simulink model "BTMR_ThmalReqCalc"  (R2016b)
settings: Solver=FixedStepDiscrete  StartTime=0.0  StopTime=10.0  FixedStep=0.1  RelTol=1e-3  EnableMultiTasking=on
undefined symbols (not defined in the file or in its folder): BMS_cntThmStbNum_C, BTMR_cntThmalReqVal_C, BTMR_flgCoolPwrCal_C, BTMR_pChrgClntPwrLv1_C, BTMR_pChrgClntPwrLv2_C, BTMR_pChrgClntPwrLv3_C, BTMR_pChrgClntPwrLv4_C, BTMR_pChrgClntPwrLv5_C, BTMR_pChrgClntPwrLv6_C, BTMR_pCoolPwrVal_C, BTMR_pHtgACPwrReq_C, BTMR_pHtgDCPwrReq_C, BTMR_pHtgDrvPwrReq_C, BTMR_pHtgsStage1_CUR, BTMR_pHtgsStage2_CUR, BTMR_pNormClntPwrLv1_C, BTMR_pNormClntPwrLv2_C, BTMR_pNormClntPwrLv3_C, BTMR_r861BrsDrvSoc_C, BTMR_r861HtgDrvSoc_C, BTMR_r891BrsDrvSoc_C, BTMR_r891HtgDrvSoc_C, BTMR_rCoolClbFlg_C, BTMR_rFlashClbFlg_C, BTMR_rHeatClbFlg_C, BTMR_t861BrsDiffLv0Temp_C, BTMR_t861BrsDiffLv1Temp_C, BTMR_t861CoolChrgAces2Temp_C, BTMR_t861CoolChrgAces3Temp_C, BTMR_t861CoolChrgAcesTemp_C, BTMR_t861CoolChrgDiffDebTemp_C, BTMR_t861CoolChrgEndDiffTemp_C, BTMR_t861CoolChrgExitLv2Temp_C, BTMR_t861CoolChrgExitLv3Temp_C, BTMR_t861CoolChrgExitTemp_C, BTMR_t861CoolChrgIntLv0Temp_C, BTMR_t861CoolChrgIntLv1Temp_C, BTMR_t861CoolChrgIntLv2Temp_C, BTMR_t861CoolChrgIntLv3Temp_C, BTMR_t861CoolChrgIntLv4Temp_C, BTMR_t861CoolChrgIntLv5Temp_C, BTMR_t861CoolDCDebTemp_C, BTMR_t861CoolNormAcesTemp_C, BTMR_t861CoolNormDiffDebTemp_C, BTMR_t861CoolNormEndDiffTemp_C, BTMR_t861CoolNormExitLv2Temp_C, BTMR_t861CoolNormExitLv3Temp_C, BTMR_t861CoolNormExitTemp_C, BTMR_t861CoolNormIntLv0Temp_C, BTMR_t861CoolNormIntLv1Temp_C, BTMR_t861CoolNormLv2Temp_C, BTMR_t861CoolNormLv3Temp_C, BTMR_t861HtgACDiffDebTemp_C, BTMR_t861HtgACEndDiffTemp_C, BTMR_t861HtgACStartHiTemp_C, BTMR_t861HtgACStartLoTemp_C, BTMR_t861HtgACStopTemp_C, BTMR_t861HtgDCDiffDebTemp_C, BTMR_t861HtgDCEndDiffTemp_C, BTMR_t861HtgDCIntLv0Temp_C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
libraries: AIWAYS_Powertrain_BMS_lib x78, simulink x9
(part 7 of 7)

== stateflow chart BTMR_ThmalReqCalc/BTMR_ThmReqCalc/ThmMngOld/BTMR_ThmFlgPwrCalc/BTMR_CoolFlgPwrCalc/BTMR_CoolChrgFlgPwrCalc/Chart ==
  state CoolChrgDefault
    en:
    BTMR_stsClntStg=enmThmCoolChrgStg_861.Default;
  state CoolChrgStage1
    state CoolChrgStage1Norm
      en:
      BTMR_stsClntStg=enmThmCoolChrgStg_861.Stg_Lv1Res;
    state CoolChrgStage1Reduce
      en:
      BTMR_stsClntStg=enmThmCoolChrgStg_861.Stg_Lv1Red;
    (default) -> CoolChrgStage1Norm
    CoolChrgStage1Norm -> CoolChrgStage1Reduce : [ CoolChrgStage1PowRed ]
    CoolChrgStage1Reduce -> CoolChrgStage1Norm : [ CoolChrgStage1PowRes ]
  state CoolChrgStage2
    state CoolChrgStage2Norm
      en:
      BTMR_stsClntStg=enmThmCoolChrgStg_861.Stg_Lv2Res;
    state CoolChrgStage2Reduce
      en:
      BTMR_stsClntStg=enmThmCoolChrgStg_861.Stg_Lv2Red;
    (default) -> CoolChrgStage2Norm
    CoolChrgStage2Norm -> CoolChrgStage2Reduce : [ CoolChrgStage2PowRed ]
    CoolChrgStage2Reduce -> CoolChrgStage2Norm : [ CoolChrgStage2PowRes ]
  state CoolChrgStage3
    state CoolChrgStage3Norm
      en:
      BTMR_stsClntStg=enmThmCoolChrgStg_861.Stg_Lv3Res;
    state CoolChrgStage3Reduce
      en:
      BTMR_stsClntStg=enmThmCoolChrgStg_861.Stg_Lv3Red;
    (default) -> CoolChrgStage3Norm
    CoolChrgStage3Norm -> CoolChrgStage3Reduce : [ CoolChrgStage3PowRed ]
    CoolChrgStage3Reduce -> CoolChrgStage3Norm : [ CoolChrgStage3PowRes ]
  (default) -> CoolChrgDefault
  CoolChrgDefault -> CoolChrgStage1
  CoolChrgStage1 -> CoolChrgStage2 : [ CoolChrgStage2Ena ]
  CoolChrgStage2 -> CoolChrgStage1 : [ CoolChrgStage2Ext ]
  CoolChrgStage2 -> CoolChrgStage3 : [ CoolChrgStage3Ena ]
  CoolChrgStage3 -> CoolChrgStage2 : [ CoolChrgStage3Ext ]
  data: CoolChrgStage2Ena input; CoolChrgStage3Ena input; BTMR_stsClntStg output Enum: enmThmCoolChrgStg_861; BTMR_pChrgClntPwrLv1_C parameter; BTMR_pChrgClntPwrLv2_C parameter; BTMR_pChrgClntPwrLv3_C parameter; CoolChrgStage2Ext input; CoolChrgStage3Ext input; CoolChrgStage1PowRed input; CoolChrgStage1PowRes input; CoolChrgStage2PowRed input; CoolChrgStage2PowRes input; CoolChrgStage3PowRed input; CoolChrgStage3PowRes input; BTMR_pChrgClntPwrLv4_C parameter; BTMR_pChrgClntPwrLv5_C parameter; BTMR_pChrgClntPwrLv6_C parameter

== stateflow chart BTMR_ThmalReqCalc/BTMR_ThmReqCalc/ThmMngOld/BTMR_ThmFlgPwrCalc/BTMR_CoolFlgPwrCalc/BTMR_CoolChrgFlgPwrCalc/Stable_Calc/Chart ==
  state Default_Stt
    en:
    i=uint8(0);
    flg_out=false;
  state AddCourse_Stt
    en:
    flg_out=true;
    du:
    i = i + uint8(1);
  (default) -> Default_Stt
  AddCourse_Stt -> Default_Stt : [ i>cntStable ]
  Default_Stt -> AddCourse_Stt : [ trigger_in==true ]
  data: i local uint8; trigger_in input boolean; flg_out output boolean; cntStable input

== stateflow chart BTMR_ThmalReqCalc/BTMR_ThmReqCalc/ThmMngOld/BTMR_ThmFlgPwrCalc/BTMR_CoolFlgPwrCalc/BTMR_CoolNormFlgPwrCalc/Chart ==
  state CoolNormDefault
    en:
    BTMR_stsClntStg=enmThmCoolNormStg_861.Default;
  state CoolNormStage1
    state CoolNormStage1Start
      en:
      BTMR_stsClntStg=enmThmCoolNormStg_861.Stg_Lv1Res;
    state CoolNormStage1Pause
      en:
      BTMR_stsClntStg=enmThmCoolNormStg_861.Stg_Lv1Red;
    (default) -> CoolNormStage1Start
    CoolNormStage1Start -> CoolNormStage1Pause : [ CoolNormPowRed ]
    CoolNormStage1Pause -> CoolNormStage1Start : [ CoolNormPowRes ]
  state CoolNormStage2
    state CoolNormStage2Start
      en:
      BTMR_stsClntStg=enmThmCoolNormStg_861.Stg_Lv2Res;
    state CoolNormStage2Pause
      en:
      BTMR_stsClntStg=enmThmCoolNormStg_861.Stg_Lv2Red;
    (default) -> CoolNormStage2Start
    CoolNormStage2Start -> CoolNormStage2Pause : [ CoolNormPowRed ]
    CoolNormStage2Pause -> CoolNormStage2Start : [ CoolNormPowRes ]
  state CoolNormStage3
    state CoolNormStage3Start
      en:
      BTMR_stsClntStg=enmThmCoolNormStg_861.Stg_Lv3Res;
    state CoolNormStage3Pause
      en:
      BTMR_stsClntStg=enmThmCoolNormStg_861.Stg_Lv3Red;
    (default) -> CoolNormStage3Start
    CoolNormStage3Start -> CoolNormStage3Pause : [ CoolNormPowRed ]
    CoolNormStage3Pause -> CoolNormStage3Start : [ CoolNormPowRes ]
  (default) -> CoolNormDefault
  CoolNormDefault -> CoolNormStage1
  CoolNormStage2 -> CoolNormStage1 : [ CoolNormStage2Ext ]
  CoolNormStage1 -> CoolNormStage2 : [ CoolNormStage2Ena ]
  CoolNormStage3 -> CoolNormStage2 : [ CoolNormStage3Ext ]
  CoolNormStage2 -> CoolNormStage3 : [ CoolNormStage3Ena ]
  data: CoolNormStage2Ena input; CoolNormStage3Ena input; BTMR_stsClntStg output Enum: enmThmCoolNormStg_861; CoolNormStage2Ext input; CoolNormStage3Ext input; CoolNormPowRed input; CoolNormPowRes input

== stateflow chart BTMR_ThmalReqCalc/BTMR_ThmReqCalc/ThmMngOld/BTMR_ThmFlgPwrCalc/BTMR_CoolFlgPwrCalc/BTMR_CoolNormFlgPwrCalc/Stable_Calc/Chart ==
  state Default_Stt
    en:
    i=uint8(0);
    flg_out=false;
  state AddCourse_Stt
    en:
    flg_out=true;
    du:
    i = i + uint8(1);
  (default) -> Default_Stt
  AddCourse_Stt -> Default_Stt : [ i>cntStable ]
  Default_Stt -> AddCourse_Stt : [ trigger_in==true ]
  data: i local uint8; trigger_in input boolean; flg_out output boolean; cntStable input

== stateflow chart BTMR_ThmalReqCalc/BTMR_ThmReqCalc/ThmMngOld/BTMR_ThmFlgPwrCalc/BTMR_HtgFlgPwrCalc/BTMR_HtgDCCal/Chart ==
  state HtgDCDefault
    en:
    BTMR_stsHeatStg=enmThmDCHeatStg_861.Default;
  state HtgDCStage1
    en:
    BTMR_stsHeatStg=enmThmDCHeatStg_861.Stg_Lv1;
  state HtgDCStage2
    state HtgDCStage2Pause
      en:
      BTMR_stsHeatStg=enmThmDCHeatStg_861.Stg_Lv2Red;
    state HtgDCStage2Curve1
      en:
      BTMR_stsHeatStg=enmThmDCHeatStg_861.Stg_Lv2Res;
    (default) -> HtgDCStage2Pause
    HtgDCStage2Pause -> HtgDCStage2Curve1 : [ HtgDCStage2PowRes ]
    HtgDCStage2Curve1 -> HtgDCStage2Pause : [ HtgDCStage2PowRed ]
  (default) -> HtgDCDefault
  HtgDCDefault -> HtgDCStage1
  (junction 44) -> HtgDCStage1
  (junction 41) -> (junction 44)
  HtgDCStage1 -> HtgDCStage2 : [ HtgDCStage2Ena ]
  HtgDCStage2 -> (junction 41) : [HtgDCStage3PowRed]
  data: HtgDCStage2Ena input; HtgDCStage2PowRed input; BTMR_stsHeatStg output Enum: enmThmDCHeatStg_861; HtgDCStage2PowRes input; HtgDCStage3PowRed input

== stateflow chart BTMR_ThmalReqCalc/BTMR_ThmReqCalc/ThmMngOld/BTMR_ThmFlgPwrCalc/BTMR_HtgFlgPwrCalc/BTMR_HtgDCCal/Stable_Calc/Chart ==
  state Default_Stt
    en:
    i=uint8(0);
    flg_out=false;
  state AddCourse_Stt
    en:
    flg_out=true;
    du:
    i = i + uint8(1);
  (default) -> Default_Stt
  AddCourse_Stt -> Default_Stt : [ i>cntStable ]
  Default_Stt -> AddCourse_Stt : [ trigger_in==true ]
  data: i local uint8; trigger_in input boolean; flg_out output boolean; cntStable input

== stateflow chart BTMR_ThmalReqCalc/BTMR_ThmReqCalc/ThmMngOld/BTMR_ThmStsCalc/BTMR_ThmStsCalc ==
  state Default_Stt
    en:
    stHtgSts=enmThmHeatSts.InActive;
    stCoolSts=enmThmCoolSts.InActive;
    stBrsSts=enmThmBrsSts.INACTIVE;
  state HtgDC_Stt
    en:
    stHtgSts=enmThmHeatSts.HeatDC;
    stCoolSts=enmThmCoolSts.InActive;
    stBrsSts=enmThmBrsSts.INACTIVE;
  state Standby_Stt
    en:
    Local_DebCnt=uint16(0);
    stHtgSts=enmThmHeatSts.InActive;
    stCoolSts=enmThmCoolSts.InActive;
    stBrsSts=enmThmBrsSts.INACTIVE;
    du:
    (default) -> (junction 139)
    Standby_Stt -> (junction 139)
    (junction 139) -> (junction 140) : [Local_DebCnt<=uint16(600)]
    (junction 139) -> (junction 141) : {Local_DebCnt=uint16(600);}
    (junction 140) -> (junction 142) : {Local_DebCnt++;}
    (junction 142) -> (junction 141)
    (junction 141) -> (junction 143)
  state CoolChrg_Stt
    en:
    stHtgSts=enmThmHeatSts.InActive;
    stCoolSts=enmThmCoolSts.CoolChrg;
    stBrsSts=enmThmBrsSts.INACTIVE;
  state HtgAC_Stt
    en:
    stHtgSts=enmThmHeatSts.HeatAC;
    stCoolSts=enmThmCoolSts.InActive;
    stBrsSts=enmThmBrsSts.INACTIVE;
  state CoolNorm_Stt
    en:
    stHtgSts=enmThmHeatSts.InActive;
    stCoolSts=enmThmCoolSts.CoolNorm;
    stBrsSts=enmThmBrsSts.INACTIVE;
  state HtgDrv_Stt
    en:
    stHtgSts=enmThmHeatSts.HeatDrv;
    stCoolSts=enmThmCoolSts.InActive;
    stBrsSts=enmThmBrsSts.INACTIVE;
  state Brush_Stt
    en:
    stHtgSts=enmThmHeatSts.InActive;
    stCoolSts=enmThmCoolSts.InActive;
    stBrsSts=enmThmBrsSts.ACTIVE;
  (default) -> Default_Stt
  Default_Stt -> Standby_Stt
  Standby_Stt -> HtgDC_Stt : [ HtgDCEna &&...  (HtgDCThmEnd==false)&&... Local_DebCnt>=uint16(600) ]
  Standby_Stt -> CoolChrg_Stt : [ CoolChrgEna &&...  (CoolChrgThmEnd==false)&&... Local_DebCnt>=uint16(600) ]
  HtgDC_Stt -> Standby_Stt : [ HtgDCThmEnd... || HtgDCDna ]
  CoolChrg_Stt -> Standby_Stt : [ CoolChrgThmEnd... || CoolChrgDna ]
  Standby_Stt -> HtgAC_Stt : [ HtgACEna &&...  (HtgACThmEnd==false)&&... Local_DebCnt>=uint16(600) ]
  HtgAC_Stt -> Standby_Stt : [ HtgACThmEnd... || HtgACDna ]
  Standby_Stt -> CoolNorm_Stt : [ CoolNormEna &&...  (CoolNormThmEnd==false)&&... Local_DebCnt>=uint16(600) ]
  Standby_Stt -> HtgDrv_Stt : [ HtgDrvEna &&...  (HtgDrvThmEnd==false)&&... Local_DebCnt>=uint16(600) ]
  CoolNorm_Stt -> Standby_Stt : [ CoolNormThmEnd...  || CoolNormDna ]
  HtgDrv_Stt -> Standby_Stt : [ HtgDrvThmEnd... || HtgDrvDna ]
  Standby_Stt -> Brush_Stt : [ (BrsEna && BrsStart) &&... (BrsThmEnd==false)&&... Local_DebCnt>=uint16(600)]
  Brush_Stt -> Standby_Stt : [ (BrsEna==false) ||...  (BrsThmEnd || BrsDna) ]
  data: stBrsSts output Enum: enmThmBrsSts; BrsEna input; HtgDCEna input; HtgACEna input; HtgDrvEna input; CoolNormEna input; CoolChrgEna input; BrsDna input; HtgDCDna input; HtgACDna input; HtgDrvDna input; CoolNormDna input; CoolChrgDna input; BrsThmEnd input; stHtgSts output Enum: enmThmHeatSts; stCoolSts output Enum: enmThmCoolSts; HtgDCThmEnd input; HtgACThmEnd input; HtgDrvThmEnd input; CoolNormThmEnd input; CoolChrgThmEnd input; BrsStart input; Local_DebCnt local uint16
